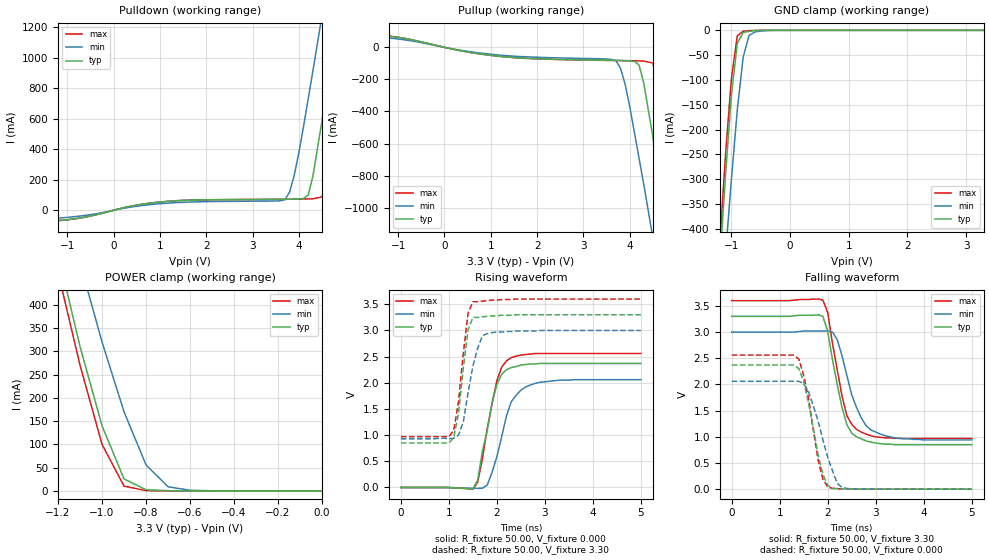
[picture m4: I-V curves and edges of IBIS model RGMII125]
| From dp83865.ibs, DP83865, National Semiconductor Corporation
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|   Model RGMII125
[Model]   RGMII125
Model_type   I/O
Polarity   Non-Inverting
Enable   Active-High
Vinl =   0.80V
Vinh =   2.00V
Vmeas =   1.50V
Cref =  20.00pF
Rref = 100.00k
C_comp   5.00pF   5.00pF   5.00pF
[Temperature Range]   25.00   0.14k   0.000
[Voltage Range]   3.30V   3.00V   3.60V
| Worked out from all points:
|   slope of the pulldown table from 0 to 0.495 V, typ, clamps not added: 14.7 ohm
|   slope of the pullup table from 0 to 0.495 V, typ, clamps not added: 17.2 ohm
|   GND clamp passes 1 mA (typ) near -0.62 V on its own axis
|   POWER clamp passes 1 mA (typ) near -0.72 V on its own axis
|   rising waveform, R_fixture 50.00, V_fixture 0.000: 20-80 % time 319ps typ, 366ps min, 314ps max; typ from 0 V to 2.37 V
|   rising waveform, R_fixture 50.00, V_fixture 3.30: 20-80 % time 188ps typ, 261ps min, 192ps max; typ from 0.85 V to 3.3 V
|   falling waveform, R_fixture 50.00, V_fixture 3.30: 20-80 % time 329ps typ, 421ps min, 324ps max; typ from 3.3 V to 0.85 V
|   falling waveform, R_fixture 50.00, V_fixture 0.000: 20-80 % time 309ps typ, 398ps min, 285ps max; typ from 2.37 V to 0 V
[Pulldown]
| voltage   I(typ)   I(min)   I(max)
-3.3V     -89.91mA   -76.56mA   -93.13mA
-1V       -61.93mA   -46.66mA   -63.1mA
1.2V      59.47mA    47.45mA    59.1mA
3.7V      72.36mA    69.99mA    71.87mA
3.9V      73.37mA    230mA      72.58mA
4.2V      100mA      730mA      74.31mA
4.3V      220mA      910mA      75.21mA
4.5V      590mA      1.28A      87.5mA
4.7V      1A         1.66A      350mA
4.9V      1.42A      2.04A      760mA
5.1V      1.85A      2.43A      1.19A
6.6V      5.19A      5.43A      4.58A
[Pullup]
| voltage   I(typ)   I(min)   I(max)
-3.3V     100mA      91.31mA    110mA
-1.5V     79.4mA     67.53mA    81.97mA
1.3V      -58.96mA   -51mA      -59.25mA
3.7V      -81.52mA   -82.85mA   -82.27mA
3.9V      -83.1mA    -230mA     -83.06mA
4.2V      -110mA     -690mA     -84.55mA
4.3V      -220mA     -850mA     -85.62mA
4.5V      -560mA     -1.19A     -97.65mA
4.7V      -930mA     -1.54A     -340mA
4.9V      -1.32A     -1.89A     -720mA
5.1V      -1.71A     -2.25A     -1.11A
6.6V      -4.85A     -5.04A     -4.3A
[GND_clamp]
| voltage   I(typ)   I(min)   I(max)
-3.3V     -4.6A      -4.3A      -4.67A
-1.2V     -470mA     -610mA     -430mA
-1.1V     -290mA     -450mA     -250mA
-1V       -130mA     -300mA     -96.48mA
-900mV    -26.18mA   -160mA     -11.2mA
-800mV    -4.33mA    -53.85mA   -1.86mA
-700mV    -1.97mA    -10.45mA   -630uA
-600mV    -770uA     -3.3mA     -120uA
-500mV    -170uA     -1.53mA    -11.66uA
-200mV    -41.47nA   -16.34uA   -920pA
3.3V      170pA      10.38uA    37.9pA
[POWER_clamp]
| voltage   I(typ)   I(min)   I(max)
-3.3V     5.01A      4.69A      5.08A
-1.2V     510mA      660mA      470mA
-1.1V     310mA      490mA      270mA
-1V       140mA      320mA      100mA
-900mV    25.8mA     170mA      10.3mA
-800mV    2.47mA     55.78mA    680uA
-700mV    550uA      8.85mA     86.56uA
-600mV    98.6uA     1.5mA      9.37uA
0V        170pA      380nA      44.23pA
[Ramp]
| variable   typ   min   max
dV/dt_r   1.92/0.12n   1.74/0.14n   2.09/0.12n
dV/dt_f   1.93/96.46p   1.74/0.12n   2.11/97.61p
R_load = 0.50k
[Rising Waveform]
R_fixture = 50.00
V_fixture = 0.000
V_fixture_min = 0.000
V_fixture_max = 0.000
| time   V(typ)   V(min)   V(max)
0s        1.14nV     480nV      920pV
1.5ns     -26.62mV   -15.79mV   -32.45mV
1.6ns     140mV      -17.39mV   100mV
1.8ns     1.09V      47.43mV    1.13V
1.9ns     1.63V      290mV      1.6V
2ns       1.97V      590mV      2.04V
2.1ns     2.16V      970mV      2.3V
2.3ns     2.29V      1.64V      2.48V
2.9ns     2.37V      2.01V      2.56V
5ns       2.37V      2.06V      2.56V
[Rising Waveform]
R_fixture = 50.00
V_fixture = 3.30
V_fixture_min = 3.00
V_fixture_max = 3.60
| time   V(typ)   V(min)   V(max)
0s        850mV      930mV      970mV
1ns       850mV      930mV      970mV
1.1ns     950mV      940mV      1.09V
1.2ns     1.41V      1V         1.63V
1.3ns     2.28V      1.25V      2.56V
1.4ns     3.01V      1.81V      3.33V
1.5ns     3.25V      2.32V      3.55V
1.7ns     3.26V      2.9V       3.56V
1.9ns     3.28V      2.96V      3.58V
5ns       3.3V       3V         3.6V
[Falling Waveform]
R_fixture = 50.00
V_fixture = 3.30
V_fixture_min = 3.00
V_fixture_max = 3.60
| time   V(typ)   V(min)   V(max)
0s        3.3V       3V         3.6V
1.9ns     3.3V       3.02V      3.61V
2ns       3.01V      3.02V      3.37V
2.2ns     1.99V      2.85V      2.27V
2.3ns     1.55V      2.54V      1.77V
2.4ns     1.23V      2.17V      1.4V
2.6ns     1V         1.56V      1.14V
2.8ns     920mV      1.21V      1.05V
3.2ns     860mV      1.02V      980mV
5ns       850mV      940mV      970mV
[Falling Waveform]
R_fixture = 50.00
V_fixture = 0.000
V_fixture_min = 0.000
V_fixture_max = 0.000
| time   V(typ)   V(min)   V(max)
0s        2.37V      2.06V      2.56V
1.4ns     2.3V       2.06V      2.48V
1.5ns     2.05V      2.01V      2.17V
1.6ns     1.65V      1.86V      1.74V
1.8ns     650mV      1.3V       560mV
1.9ns     280mV      940mV      190mV
2ns       74.06mV    610mV      42.18mV
2.2ns     9.96mV     110mV      9.29mV
2.3ns     6.99mV     30.92mV    6.47mV
5ns       -6.27uV    16.52uV    -49.06nV
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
